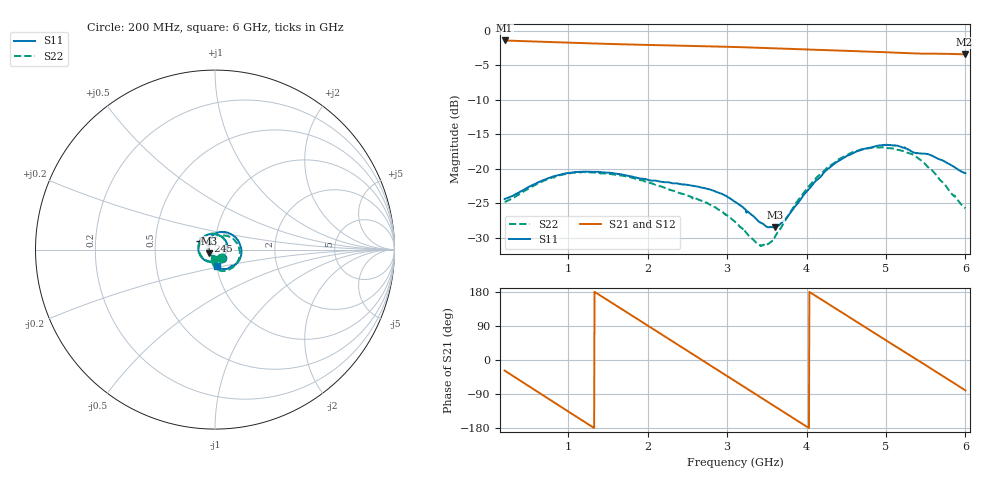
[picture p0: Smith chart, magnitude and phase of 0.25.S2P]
!Agilent Technologies,E5071C,MY46316741,A.11.02
!Date: Fri Apr 15 16:18:43 2022
!Data & Calibration Information:
!Freq	S11:SOLT2(ON)	S21:SOLT2(ON)	S12:SOLT2(ON)	S22:SOLT2(ON)
!PortZ  Port1:50+j0  Port2:50+j0
!Above PortZ is port z conversion or system Z0 setting when saving the data.
!When reading, reference impedance value at option line is always used.
# Hz S dB R 50
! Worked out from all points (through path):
!   1200 points, 200 MHz to 6 GHz, reference 50 ohm
!   highest |S21| = -1.38 dB at 200 MHz (marker M1); lowest = -3.4 dB at 5.99 GHz (marker M2)
!   group delay of S21, straight-line fit = 370 ps
!   lowest |S11| = -28.5 dB at 3.606 GHz (marker M3), VSWR 1.08, Z = 46.9 - j1.87 ohm
!   |S11| at or under -10 dB: start of sweep to end of sweep
!   |S22| runs from -31.2 to -16.9 dB; largest |S21 - S12| = 0.0026
!   S11 on the Smith chart (normalised r, x): 200 MHz: 1.08, -0.10; 1.245 GHz: 0.84, +0.08; 6 GHz: 1.00, -0.19
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2e8  -24.39 -49.3  -1.38 -27.9  -1.38 -27.9  -24.84 -52.6
4.563803e8  -22.96 -98.3  -1.49 -62.6  -1.49 -62.6  -23.18 -104.6
6.740617e8  -21.73 -133.9  -1.57 -92.0  -1.57 -92.0  -21.87 -142.2
9.014178e8  -20.86 -166.4  -1.66 -122.5  -1.66 -122.5  -20.94 -176.5
1.167473e9  -20.45 159.9  -1.76 -158.2  -1.76 -158.1  -20.51 147.7
1.244871e9  -20.42 150.8  -1.79 -168.5  -1.79 -168.5  -20.51 137.9
1.481902e9  -20.57 125.2  -1.88 159.9  -1.88 159.9  -20.70 110.2
1.747957e9  -21.03 99.2  -1.96 124.6  -1.96 124.6  -21.15 81.0
2.134946e9  -21.81 66.8  -2.06 73.1  -2.06 73.1  -22.49 42.7
2.401001e9  -22.22 43.9  -2.12 37.6  -2.12 37.6  -23.54 18.9
2.628357e9  -22.60 22.4  -2.19 7.3  -2.19 7.3  -24.43 -2.2
2.855713e9  -23.32 -2.5  -2.25 -23.0  -2.25 -23.0  -25.62 -27.0
3.102419e9  -24.82 -35.5  -2.33 -55.9  -2.33 -55.9  -27.73 -61.5
3.353962e9  -27.15 -80.7  -2.42 -89.5  -2.42 -89.4  -30.59 -115.8
3.605505e9  -28.51 -147.8  -2.51 -123.0  -2.51 -122.9  -29.82 165.4
3.847373e9  -25.62 148.1  -2.62 -155.2  -2.61 -155.1  -25.38 110.5
4.069892e9  -22.40 105.7  -2.72 175.2  -2.71 175.3  -22.02 75.1
4.577815e9  -17.80 36.7  -2.91 107.9  -2.91 108.0  -17.62 10.5
5.037364e9  -16.55 -14.4  -3.10 47.1  -3.11 47.2  -17.03 -41.0
5.492077e9  -17.82 -53.0  -3.29 -12.7  -3.29 -12.6  -19.30 -85.1
5.990325e9  -20.61 -83.2  -3.40 -78.9  -3.40 -78.9  -25.65 -97.6
6e9  -20.66 -83.4  -3.40 -80.2  -3.41 -80.1  -25.75 -97.1
